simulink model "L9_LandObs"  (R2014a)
settings: Solver=ode45  StartTime=0.0  StopTime=tend  RelTol=1e-3
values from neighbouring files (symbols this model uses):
  A = [0 1; 0 0]    [L9.m]    (also in L9_LandObs_script.m; L9_fullExample_script.m; L9_onlyL_script.m)
  Aob = Phi-Gamma*L-K*C    [L9_LandObs_script.m]    (also in L9_fullExample_script.m = [ Phi-Gamma*L-K*C, zeros(size(A,1),1))
  B = [0; 1]    [L9.m]    (also in L9_LandObs_script.m; L9_fullExample_script.m; L9_onlyL_script.m)
  Bob = K    [L9_LandObs_script.m]    (also in L9_fullExample_script.m = Ke)
  C = [1, 0]    [L9.m]    (also in L9_LandObs_script.m; L9_fullExample_script.m; L9_onlyL_script.m)
  Cob = eye(size(Aob))    [L9_LandObs_script.m]    (also in L9_fullExample_script.m)
  Cx = eye(size(A))    [L9.m]    (also in L9_LandObs_script.m; L9_fullExample_script.m; L9_onlyL_script.m)
  Dob = zeros(size(Cob,1),size(Bob,2))    [L9_LandObs_script.m]    (also in L9_fullExample_script.m)
  Dx = zeros(size(Cx,1),size(B,2))    [L9.m]    (also in L9_LandObs_script.m; L9_fullExample_script.m; L9_onlyL_script.m)
  h = h3    (= 0.5)    [L9.m]    (also in L9_LandObs_script.m = 0.44; L9_fullExample_script.m = 0.44; L9_onlyL_script.m = 0.44)
  L = L3    [L9.m]    (also in L9_LandObs_script.m = place(Phi,Gamma,pd); L9_fullExample_script.m = place(Phi,Gamma,pd); L9_onlyL_script.m = place(Phi,Gamma,pd))
  x0 = [1;1]    [L9.m]    (also in L9_LandObs_script.m; L9_fullExample_script.m; L9_onlyL_script.m)

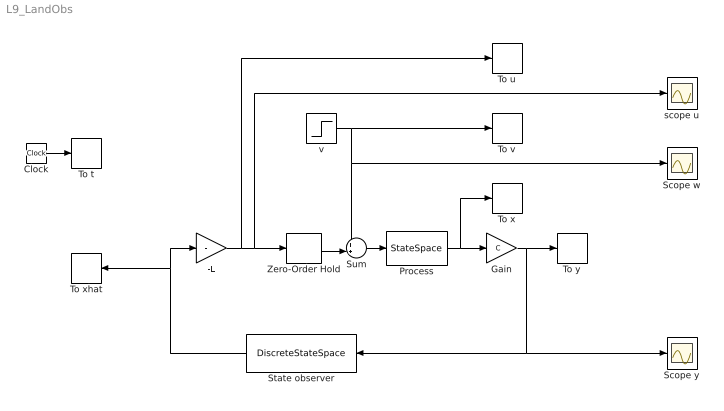
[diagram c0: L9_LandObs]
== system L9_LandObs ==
  -L : Gain  Gain=-L  Multiplication=Matrix(K*u)  SampleTime=h
  Clock : Clock
  Gain : Gain  Gain=C  Multiplication=Matrix(K*u)
  Process : StateSpace  A=A  B=B  C=Cx  D=Dx  X0=x0
  Scope w : Scope
  Scope y : Scope
  State observer : DiscreteStateSpace  A=Aob  B=Bob  C=Cob  D=Dob  SampleTime=h
  Sum : Sum  Inputs=++|
  To t : ToWorkspace  VariableName=t  SampleTime=h
  To u : ToWorkspace  VariableName=u  SampleTime=h
  To v : ToWorkspace  VariableName=v  SaveFormat=Structure With Time  SampleTime=-1
  To x : ToWorkspace  VariableName=x  SaveFormat=Structure With Time  SampleTime=-1
  To xhat : ToWorkspace  VariableName=xhat  SampleTime=h
  To y : ToWorkspace  VariableName=y  SaveFormat=Structure With Time  SampleTime=-1
  Zero-Order Hold : ZeroOrderHold  SampleTime=h
  scope u : Scope
  v : Step  Time=25  After=-0.5  SampleTime=0
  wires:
  -L/1 -> To u/1, scope u/1, Zero-Order Hold/1
  Clock/1 -> To t/1
  Process/1 -> To x/1, Gain/1
  Sum/1 -> Process/1
  Zero-Order Hold/1 -> Sum/2
  State observer/1 -> To xhat/1, -L/1
  v/1 -> Sum/1, Scope w/1, To v/1
  Gain/1 -> State observer/1, Scope y/1, To y/1
